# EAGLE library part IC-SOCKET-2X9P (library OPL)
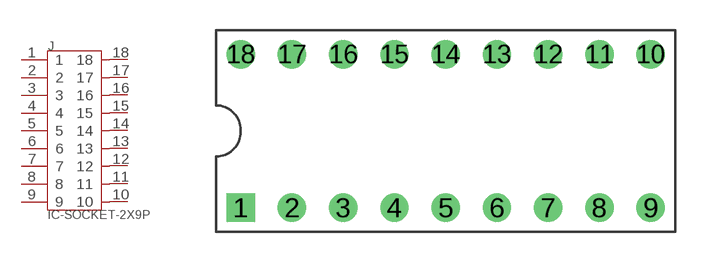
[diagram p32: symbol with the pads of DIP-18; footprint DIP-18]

Designator prefix J

## IC-SOCKET-2X9P-320070007  [DIP-18]
1  1
2  2
3  3
4  4
5  5
6  6
7  7
8  8
9  9
10  10
11  11
12  12
13  13
14  14
15  15
16  16
17  17
18  18

## Footprint DIP-18 (pad centres in mm)
drill 0.9 pad 1.4 square: 1 -10.16,-3.81
drill 0.9 pad 1.4: 2 -7.62,-3.81; 3 -5.08,-3.81; 4 -2.54,-3.81; 5 0,-3.81; 6 2.54,-3.81; 7 5.08,-3.81; 8 7.62,-3.81; 9 10.16,-3.81; 10 10.16,3.81; 11 7.62,3.81; 12 5.08,3.81; 13 2.54,3.81; 14 0,3.81; 15 -2.54,3.81; 16 -5.08,3.81; 17 -7.62,3.81; 18 -10.16,3.81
